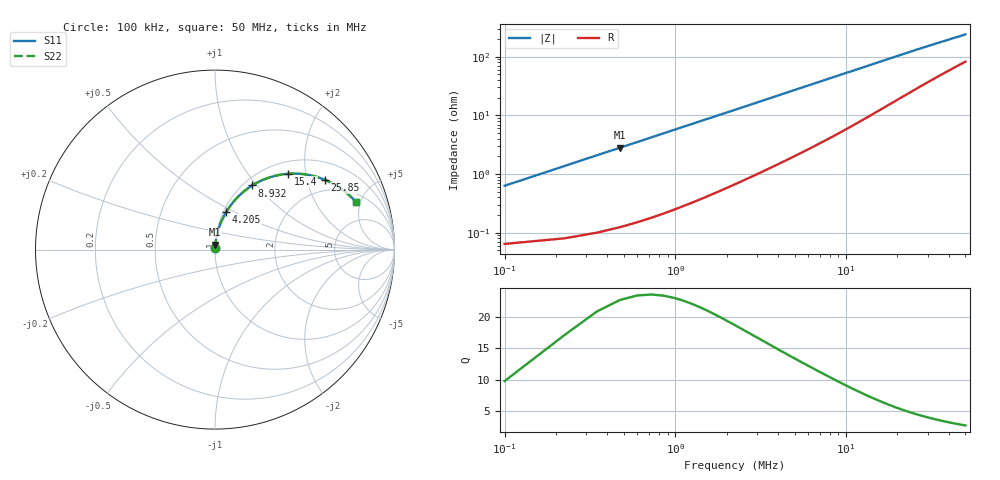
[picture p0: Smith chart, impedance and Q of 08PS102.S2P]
! Coilcraft 0805PS-102 Power Chip Inductor
! 5 February 2003
# MHZ S MA R 50
!Freq  MagS11  AngS11  MagS21  AngS21  MagS12  AngS12  MagS22  AngS22
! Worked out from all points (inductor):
!   403 points, 100 kHz to 50 MHz, reference 50 ohm
!   read as one part in series: L = 944 nH near 348.8 kHz
!   highest Q = 22.6 at 473.2 kHz (marker M1), where L = 944 nH
!   S11 on the Smith chart (normalised r, x): 100 kHz: 1.00, +0.01; 4.205 MHz: 1.03, +0.46; 8.932 MHz: 1.10, +0.95; 15.4 MHz: 1.24, +1.59; 25.85 MHz: 1.57, +2.58; 50 MHz: 2.65, +4.52
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0.1  0.006311 83.8  0.9993 -0.4  0.9993 -0.4  0.006311 83.8
0.2244  0.0137 85.9  0.9991 -0.8  0.9991 -0.8  0.0137 85.9
0.4732  0.02805 85.9  0.9984 -1.6  0.9984 -1.6  0.02805 85.9
0.5976  0.03509 85.5  0.9979 -2.0  0.9979 -2.0  0.03509 85.5
0.722  0.04206 85.2  0.9973 -2.4  0.9973 -2.4  0.04206 85.2
0.9708  0.05583 84.3  0.996 -3.2  0.996 -3.2  0.05583 84.3
1.344  0.07612 83.0  0.9936 -4.4  0.9936 -4.4  0.07612 83.0
1.7172  0.09604 81.7  0.9907 -5.5  0.9907 -5.5  0.09604 81.7
2.2148  0.1221 79.9  0.986 -7.0  0.986 -7.0  0.1221 79.9
2.8368  0.1538 77.8  0.9792 -8.8  0.9792 -8.8  0.1538 77.8
4.2052  0.2203 73.4  0.9604 -12.7  0.9604 -12.7  0.2203 73.4
6.0712  0.3035 67.7  0.9282 -17.6  0.9282 -17.6  0.3035 67.7
8.4348  0.3957 61.2  0.8802 -23.2  0.8802 -23.2  0.3957 61.2
8.9324  0.4132 59.9  0.8694 -24.3  0.8694 -24.3  0.4132 59.9
11.918  0.5051 52.9  0.8032 -30.1  0.8032 -30.1  0.5051 52.9
15.4012  0.5868 46.0  0.7279 -35.5  0.7279 -35.5  0.5868 46.0
16.7696  0.6127 43.7  0.7 -37.2  0.7 -37.2  0.6127 43.7
25.1044  0.7189 33.1  0.5593 -44.6  0.5593 -44.6  0.7189 33.1
25.8508  0.7254 32.4  0.549 -45.1  0.549 -45.1  0.7254 32.4
33.4392  0.7746 26.5  0.4618 -48.4  0.4618 -48.4  0.7746 26.5
41.774  0.8073 22.0  0.3934 -50.3  0.3934 -50.3  0.8073 22.0
50  0.828 18.9  0.3443 -51.0  0.3443 -51.0  0.828 18.9
